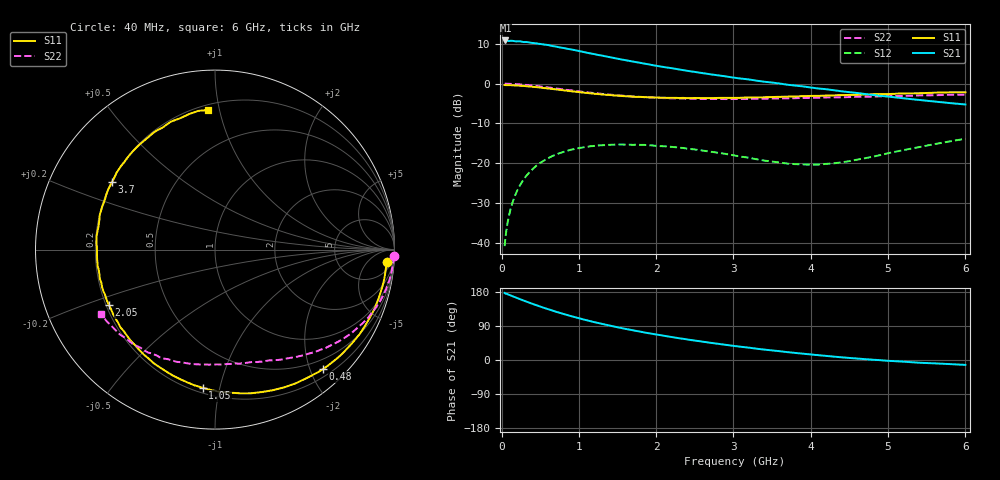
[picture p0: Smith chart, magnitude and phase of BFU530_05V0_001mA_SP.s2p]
! Filename:  P:\Prog\Test\Noise\ATS_data\Testdata_Net\03 Spar\BFU530_APG2013_40_A05_05p0V_001mA_SP_CM01_D.s2p
! Date/Time: Fri 26/Apr/2013 13:03:16
! BFU530_APG2013_40_A05_05p0V_1to25mA_SP_CM01_Bias1_R.s2p
! MDIF S-parameter v. bias file
! BFU530_APG2013_40_A05_05p0V_1to25mA_SP_CM01
! Date/time Wed Apr 24 19:36:53 2013
! bias mode 1
! bias variable = I_out
! VAR bias_var= 1
! VAR V_out= 5.0000
! VAR I_out= 0.9950
! VAR V_in= 0.7821
! VAR I_in= 0.0105
! Device data file deembeded for feedlines and parallel
! Original file: \03 Spar\BFU530_APG2013_40_A05_05p0V_001mA_SP_CM01_R.s2p
! Feed-files: PR047V01_250413_Feed1.s2p, PR047V01_250413_Feed2.s2p
! Parallel-file: PR047V01_250413_Par.s2p
# MHz S MA R 50
!  Freq-MHz  S11-mag  S11-arg  S21-mag  S21-arg  S12-mag  S12-arg  S22-mag  S22-arg
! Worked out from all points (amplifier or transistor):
!   98 points, 40 MHz to 6 GHz, reference 50 ohm
!   highest |S21| = 10.9 dB at 50 MHz (marker M1)
!   |S21| within 3 dB of that: start of sweep to 1.085 GHz
!   unconditionally stable (mu >= 1): 3.275 GHz to 4.999 GHz
!   at 300 MHz: K = 0.09, MSG = 17.1 dB, |S12| = -23.7 dB
!   at 1.6 GHz: K = 0.41, MSG = 10.6 dB, |S12| = -15.3 dB
!   at 6 GHz: K = 0.80, MSG = 4.3 dB, |S12| = -13.9 dB
!   S11 on the Smith chart (normalised r, x): 40 MHz: 12, -21; 480 MHz: 0.32, -2.21; 1.05 GHz: 0.23, -0.89; 2.05 GHz: 0.21, -0.23; 3.7 GHz: 0.20, +0.29; 6 GHz: 0.23, +0.92
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40  0.9608 -4.1  3.476 177.0  0.009072 87.0  0.9971 -2.1
50  0.9588 -5.1  3.487 175.4  0.01137 86.5  0.9969 -2.7
100  0.957 -10.2  3.433 171.8  0.02269 83.2  0.9938 -5.5
120  0.9553 -12.3  3.46 170.2  0.02714 81.9  0.992 -6.6
200  0.948 -20.4  3.392 163.7  0.04467 76.4  0.9829 -11.1
240  0.9409 -24.6  3.401 160.4  0.05304 73.8  0.9776 -13.2
340  0.9248 -34.5  3.317 152.7  0.07289 67.4  0.9578 -18.5
480  0.8976 -47.9  3.164 142.5  0.09765 59.0  0.9263 -25.2
600  0.87 -58.9  3.059 134.3  0.1155 52.4  0.8958 -30.6
700  0.8469 -67.7  2.929 127.7  0.1278 47.2  0.8704 -34.7
900  0.8015 -83.8  2.687 115.8  0.148 38.1  0.8235 -41.9
1050  0.7726 -95.1  2.511 107.5  0.1577 31.9  0.7878 -46.9
1250  0.7395 -108.7  2.291 97.7  0.1671 24.8  0.7528 -52.4
1500  0.7067 -124.2  2.058 86.4  0.1716 16.9  0.7142 -59.1
1750  0.6817 -138.1  1.856 76.4  0.1707 10.4  0.684 -65.0
2050  0.667 -152.6  1.645 65.7  0.1641 4.2  0.6602 -71.5
2500  0.6604 -171.8  1.403 51.3  0.1489 -2.5  0.6445 -80.8
3100  0.6646 165.9  1.157 34.9  0.121 -4.2  0.6416 -92.9
3700  0.6861 146.6  0.9683 20.8  0.09884 5.1  0.6535 -105.1
4100  0.7029 135.6  0.8683 12.7  0.09628 17.6  0.6643 -113.2
5200  0.7542 109.0  0.6539 -4.4  0.1463 38.8  0.7004 -135.0
6000  0.7789 92.9  0.5473 -12.9  0.203 37.0  0.7282 -150.4
